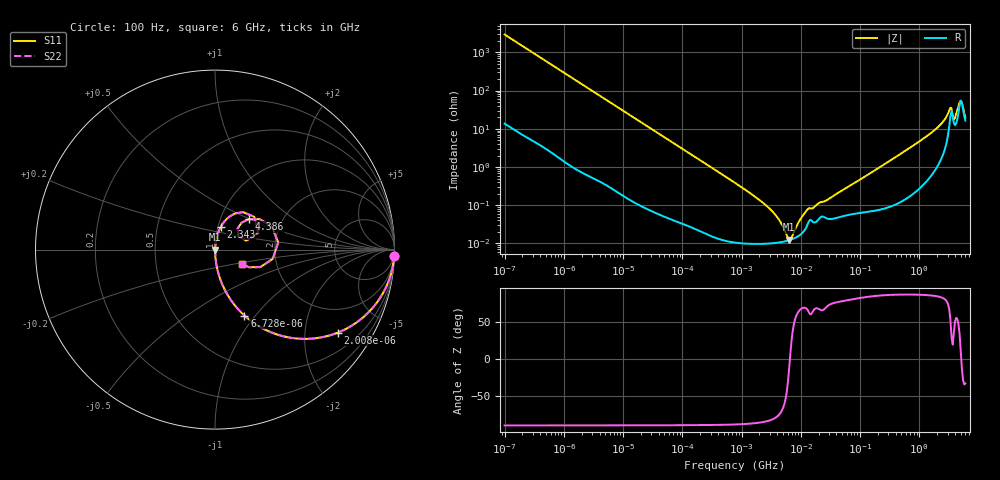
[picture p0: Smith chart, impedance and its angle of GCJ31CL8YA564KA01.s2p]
!Murata Part Number: GCJ31CL8YA564KA01
!These Parameters are Measured in Series Mode Connection
!Data Generated on Mar 13, 2026
!  o--ll--o
!Port1  Port2
!  o------o
!Operation Temp=25[degC], DC Bias Voltage=0[V]
!Freq. Start=100[Hz] Stop=6[GHz] 401[Steps]
# Hz S RI R 50
!Freq.(Hz) S11(Real) S11(Imag) S21(Real) S21(Imag) S12(Real) S12(Imag) S22(Real) S22(Imag)
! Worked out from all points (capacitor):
!   401 points, 100 Hz to 6 GHz, reference 50 ohm
!   read as one part in series: C = 543 nF near 109 Hz
!   lowest |Z| = 12.5 mohm at 6.353 MHz (marker M1)
!   series resonance near 6.549 MHz, so ESL is about 1.1 nH
!   S11 on the Smith chart (normalised r, x): 100 Hz: 1, -59; 2.008 kHz: 1.01, -2.94; 6.728 kHz: 1.01, -0.88; 2.343 GHz: 1.03, +0.27; 4.386 GHz: 1.36, +0.50; 6 GHz: 1.33, -0.21
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100  0.9987 -0.0341  0.00133 0.0341  0.00133 0.0341  0.9987 -0.0341
717  0.943 -0.2294  0.057 0.2294  0.057 0.2294  0.943 -0.2294
2008  0.6828 -0.463  0.3172 0.463  0.3172 0.463  0.6828 -0.463
3437  0.4257 -0.4917  0.5743 0.4917  0.5743 0.4917  0.4257 -0.4917
6728  0.1641 -0.3674  0.8359 0.3674  0.8359 0.3674  0.1641 -0.3674
13772  0.0456 -0.2057  0.9544 0.2057  0.9544 0.2057  0.0456 -0.2057
40335  0.006 -0.0735  0.994 0.0735  0.994 0.0735  0.006 -0.0735
774597  0.00012 -0.00385  0.9999 0.00385  0.9999 0.00385  0.00012 -0.00385
3103719  0.000101 -0.000757  0.9999 0.000757  0.9999 0.000757  0.000101 -0.000757
4246196  0.000106 -0.000414  0.9999 0.000414  0.9999 0.000414  0.000106 -0.000414
6353432  0.000122 -2.81e-05  0.9999 2.81e-05  0.9999 2.81e-05  0.000122 -2.81e-05
6948629  0.000128 5.54e-05  0.9999 -5.54e-05  0.9999 -5.54e-05  0.000128 5.54e-05
9090158  0.000156 0.000315  0.9998 -0.000315  0.9998 -0.000315  0.000156 0.000315
1.189169e7  0.000237 0.000616  0.9998 -0.000616  0.9998 -0.000616  0.000237 0.000616
1.555665e7  0.00038 0.000733  0.9996 -0.000733  0.9996 -0.000733  0.00038 0.000733
3.124326e8  0.0011 0.0142  0.9989 -0.0142  0.9989 -0.0142  0.0011 0.0142
2.34314e9  0.0327 0.1276  0.9673 -0.1276  0.9673 -0.1276  0.0327 0.1276
3.205649e9  0.1563 0.2088  0.8437 -0.2088  0.8437 -0.2088  0.1563 0.2088
4.009986e9  0.1255 0.1166  0.8745 -0.1166  0.8745 -0.1166  0.1255 0.1166
4.385646e9  0.1895 0.1708  0.8105 -0.1708  0.8105 -0.1708  0.1895 0.1708
5.016141e9  0.3521 0.0404  0.6479 -0.0404  0.6479 -0.0404  0.3521 0.0404
6e9  0.1478 -0.0784  0.8522 0.0784  0.8522 0.0784  0.1478 -0.0784
